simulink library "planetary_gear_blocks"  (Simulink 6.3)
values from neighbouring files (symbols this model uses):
  b_c = kb*J_c    (= 4.94590955184)    [architetture_epicicloidale.m]    (also in architetture_epicicloidale_cont.m; architetture_epicicloidale_HEV.m = 92.8974810391; architetture_epicicloidale_prova.m; architetture_HEV_controllo.m = 9.28974810391)
  b_p = kb*J_p    (= 8.12277148259)    [architetture_epicicloidale_HEV.m]    (also in architetture_HEV_controllo.m = 0.812277148259; architetture_HEV_startstop.m = 0.0731049433433; Confronto_CVT_EMR.m = 0; epicicloidale_confronto_statico_elastico.m)
  b_r = kb*J_r    (= 218.026030555)    [architetture_epicicloidale.m]    (also in architetture_epicicloidale_cont.m; architetture_epicicloidale_HEV.m; architetture_epicicloidale_prova.m; architetture_HEV_controllo.m = 21.8026030555)
  b_s = kb*J_s    (= 8.12277148259)    [architetture_epicicloidale.m]    (also in architetture_epicicloidale_cont.m; architetture_epicicloidale_HEV.m = 4.94590955184; architetture_epicicloidale_prova.m; architetture_HEV_controllo.m = 0.494590955184)
  d_cr = d0    (= 10)    [architetture_epicicloidale_HEV.m]    (also in architetture_HEV_controllo.m = 1000; architetture_HEV_startstop.m = 90; epicicloidale_confronto_statico_elastico.m; epicicloidale_statico.m)
  d_sc = d0    (= 10)    [architetture_epicicloidale_HEV.m]    (also in architetture_HEV_controllo.m = 1000; architetture_HEV_startstop.m = 90; epicicloidale_confronto_statico_elastico.m; epicicloidale_statico.m)
  J_c = 1.3*0.5*pi*rho_acc*hc*r_c^4    (= 0.0494590955184)    [architetture_epicicloidale.m]    (also in architetture_epicicloidale_cont.m; architetture_epicicloidale_HEV.m = 0.928974810391; architetture_epicicloidale_prova.m; architetture_HEV_controllo.m = 0.928974810391)
  J_p = Nr_sat*0.5*pi*rho_acc*(hs*r_p^4 + hc*r_p^4)    (= 0.0812277148259)    [architetture_epicicloidale_HEV.m]    (also in architetture_HEV_controllo.m; architetture_HEV_startstop.m; Confronto_CVT_EMR.m = 0; epicicloidale_confronto_statico_elastico.m)
  J_r = 0.5*pi*rho_acc*(hr*r_ri^4 + h_ring*(r_re^4-r_ri^4))    (= 2.18026030555)    [architetture_epicicloidale.m]    (also in architetture_epicicloidale_cont.m; architetture_epicicloidale_HEV.m; architetture_epicicloidale_prova.m; architetture_HEV_controllo.m)
  J_s = Nr_sat*0.5*pi*rho_acc*(hs*r_s^4 + hc*r_s^4)    (= 0.0812277148259)    [architetture_epicicloidale.m]    (also in architetture_epicicloidale_cont.m; architetture_epicicloidale_HEV.m = 0.0494590955184; architetture_epicicloidale_prova.m; architetture_HEV_controllo.m = 0.0494590955184)
  K_cr = K0    (= 10000)    [architetture_epicicloidale_HEV.m]    (also in architetture_HEV_controllo.m = 100000; architetture_HEV_startstop.m = 10000000; epicicloidale_confronto_statico_elastico.m; epicicloidale_statico.m)
  K_sc = K0    (= 10000)    [architetture_epicicloidale_HEV.m]    (also in architetture_HEV_controllo.m = 100000; architetture_HEV_startstop.m = 10000000; epicicloidale_confronto_statico_elastico.m; epicicloidale_statico.m)
  Nr_sat = 4    [architetture_epicicloidale.m]    (also in architetture_epicicloidale_cont.m; architetture_epicicloidale_HEV.m; architetture_epicicloidale_prova.m; architetture_HEV_controllo.m)
  r_p = xds*Np/(2*pi)    (= 0.0732112738223)    [architetture_epicicloidale_HEV.m]    (also in architetture_HEV_controllo.m; architetture_HEV_startstop.m; Confronto_CVT_EMR.m = 0.025; epicicloidale_confronto_statico_elastico.m)
  r_r = xds*Nr/(2*pi)    (= 0.248281711223)    [architetture_epicicloidale_HEV.m]    (also in architetture_HEV_controllo.m; architetture_HEV_startstop.m; Confronto_CVT_EMR.m = 0.1; epicicloidale_confronto_statico_elastico.m)
  r_s = xds*Ns/(2*pi)    (= 0.0732112738223)    [architetture_epicicloidale.m]    (also in architetture_epicicloidale_cont.m; architetture_epicicloidale_HEV.m = 0.101859163579; architetture_epicicloidale_prova.m; architetture_HEV_controllo.m = 0.101859163579)
  Tc = 0.05*ms    (= 5e-05)    [architetture_epicicloidale.m]    (also in architetture_epicicloidale_cont.m; architetture_epicicloidale_HEV.m; architetture_epicicloidale_prova.m; architetture_HEV_controllo.m)
  Tc_0 = 0*N*metri    (= 0)    [architetture_epicicloidale_HEV.m]    (also in architetture_HEV_controllo.m; architetture_HEV_startstop.m; epicicloidale_confronto_statico_elastico.m; epicicloidale_statico.m)
  Tr_0 = 0*N*metri    (= 0)    [architetture_epicicloidale_HEV.m]    (also in architetture_HEV_controllo.m; architetture_HEV_startstop.m; epicicloidale_confronto_statico_elastico.m; epicicloidale_statico.m)
  Ts_0 = 0*N*metri    (= 0)    [architetture_epicicloidale_HEV.m]    (also in architetture_HEV_controllo.m; architetture_HEV_startstop.m; epicicloidale_confronto_statico_elastico.m; epicicloidale_statico.m)
  Wc_0 = 0*0.1*rad/secondo    (= 0)    [architetture_epicicloidale.m]    (also in architetture_epicicloidale_cont.m; architetture_epicicloidale_HEV.m; architetture_epicicloidale_prova.m; Confronto_CVT_EMR.m)
  Wr_0 = Sys1.C(3,:)*[Wc_0; Wsc_0]    [architetture_epicicloidale.m]    (also in Confronto_CVT_EMR.m = 0; epicicloidale.m; epicicloidale_confronto_statico_elastico.m = [-r_s/r_r, 1+r_s/r_r]*[Ws_0; Wc_0]; epicicloidale_da_solo.m = [ -1/r_ri*r_c, (r_c+r_ri)/r_ri]*[Wc_0; Wsc_0])
  Ws_0 = 0.1*rad/secondo    (= 0.1)    [epicicloidale_confronto_statico_elastico.m]    (also in epicicloidale_statico.m; architetture_epicicloidale_statico.m = 0)
undefined symbols (not defined in the file or in its folder): Wr, Ws

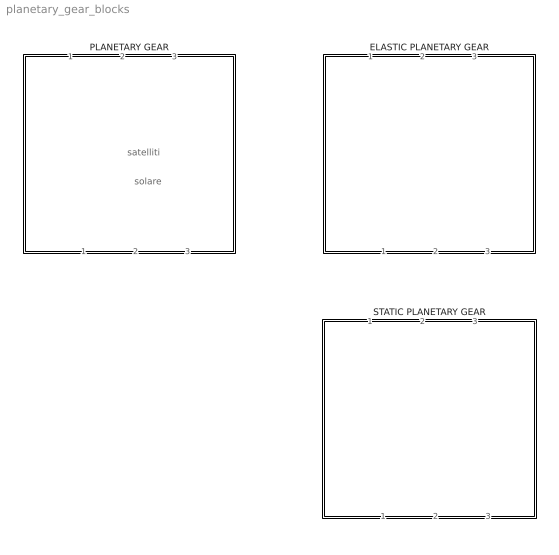
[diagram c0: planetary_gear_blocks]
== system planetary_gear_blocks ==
  note: solare
  note: satelliti
  ELASTIC PLANETARY GEAR : Subsystem  Orientation=down  mask(POG Gruppo epicicloidale){Par_solare=[J_s, b_s, r_s], Par_satelliti=[J_p, J_c, b_p, b_c, r_p, Nr_sat], Par_ring=[J_r, b_r, r_r], Solare_Satelliti=[K_sc, d_sc], Satelliti_Ring=[K_cr, d_cr], Cond_in=[Ts_0, Tc_0, Tr_0]}
      mask prompts: Par_solare "Parametri Solare: [J_s, b_s, r_s]-->[kg*m^2,N*m*s/rad,m]"; Par_satelliti "Parametri Satelliti: [J_p, J_c, b_p, b_c, r_p, Nr_sat]-->[kg*m^2,N*m*s/rad,m]"; Par_ring "Parametri Ring: [J_r, b_r, r_r]-->[kg*m^2,N*m*s/rad,m,m]"; Solare_Satelliti "Solare-Satelliti: [K_sc, d_sc]-->[N/m,N*m*s/rad]"; Satelliti_Ring "Satelliti-Ring: [K_cr, d_cr]-->[N/m,N*m*s/rad]"; Cond_in "Condizioni iniziali: [Ts_0, Tc_0, Tr_0]-->[N]"
      mask help: Gruppo epicicloidale: [J_s, J_p, J_c, J_r]= Inerzie di: solare, satelliti, porta-satelliti, ring; [b_s, b_p, b_c, b_r]= Attriti di: solare, satelliti, porta-satelliti, ring; [r_s, r_p, r_r]= Raggi di: solare, satelliti, ring; [Nr_sat]= Numero Satelliti; [K_sc, K_cr]= Elasticita' tra solare-satelliti e tra satelliti-ring; [d_sc, d_cr]= Elementi della matrice D; [Ws_0, Wc_0, Wr_0]=Velocita' iniziali di solare, porta-satelliti, ring;
      mask init:
      | J_s=double(Par_solare(1));          
      | b_s=double(Par_solare(2));            
      | r_s=double(Par_solare(3));           
      | %
      | J_p=double(Par_satelliti(1));            
      | J_c=double(Par_satelliti(2));            
      | b_p=double(Par_satelliti(3));            
      | b_c=double(Par_satelliti(4));            
      | r_p=double(Par_satelliti(5));            
      | Nr_sat=double(Par_satelliti(6));           
      | %
      | J_r=double(Par_ring(1));             
      | b_r=double(Par_ring(2));            
      | r_r=double(Par_ring(3));                  
      | %
      | %%%%%%%%%%%%%%%%%%%%%%%%%%%%%%%%%%%%%%%%%%%%%%%%%%%%%%%%%%%%%%%%%%%%%%%%%%%
      | %   Modello solo elastico
      | %%%%%%%%%%%%%%%%%%%%%%%%%%%%%%%%%%%%%%%%%%%%%%%%%%%%%%%%%%%%%%%%%%%%%%%%%%%
      |       
      |     %
      |     K_sc=double(Solare_Satelliti(1));
      |     d_sc=double(Solare_Satelliti(2));
      |     if(K_sc==0)
      |         K_sc=inf;
      |     end
      |     %
      |     K_cr=double(Satelliti_Ring(1));
      |     d_cr=double(Satelliti_Ring(2));
      |     if(K_cr==0)
      |         K_cr=inf;
      |     end
      |     
      |     %
      |     L=[1/K_sc,      0,      0;
      |             0,    J_p,      0;
      |             0,      0, 1/K_cr];
      |     %
      | 
      |     A=-[                          0,                        r_p,                          0;
      |                                -r_p, -d_sc*r_p^2-r_p^2*d_cr-b_p,                       -r_p;
      |                                   0,                        r_p,                          0];
      |        
      |     B=[                      r_s,                     -r_s,                        0;
      |                    -r_s*d_sc*r_p, -(d_cr*r_r-r_s*d_sc)*r_p,             r_p*d_cr*r_r;
      |                               0,                      r_r,                     -r_r];
      |     C=[                     r_s,            r_s*d_sc*r_p,                       0;
      |                            -r_s, (d_cr*r_r-r_s*d_sc)*r_p,                     r_r;
      |                               0,           -r_p*d_cr*r_r,                    -r_r];
      |     
      |     D= [    b_s+r_s^2*d_sc,               -r_s^2*d_sc,                         0;
      |                -r_s^2*d_sc, b_c+r_s^2*d_sc+r_r^2*d_cr,               -r_r^2*d_cr;
      |                          0,               -r_r^2*d_cr,            b_r+r_r^2*d_cr];
      |        
      |      %
      |     Ts_0=double(Cond_in(1));
      |     Tc_0=double(Cond_in(2));
      |     Tr_0=double(Cond_in(3));
      |     
      |     %
      |     We_0=[Ts_0 Tc_0 Tr_0];
  PLANETARY GEAR : Subsystem  Orientation=down  mask(POG Gruppo epicicloidale){Par_solare=[J_s, b_s, r_s], Par_satelliti=[J_p, J_c, b_p, b_c, r_p, Nr_sat], Par_ring=[J_r, b_r, r_r], Tipo_di_Modello=Modello esteso, Cond_in_Ws_Wc=[Ws_0,  Wc_0], Cond_in_Wc_Wr=[Wc_0,  Wr_0], Cond_in_Ws_Wr=[Ws_0,  Wr_0], Solare_Satelliti=[K_sc, d_sc], Satelliti_Ring=[K_cr, d_cr], Cond_in=[Ws_0, Wc_0, Wr_0]}
      mask prompts: Par_solare "Parametri Solare: [J_s, b_s, r_s]-->[kg*m^2,N*m*s/rad,m]"; Par_satelliti "Parametri Satelliti: [J_p, J_c, b_p, b_c, r_p, Nr_sat]-->[kg*m^2,N*m*s/rad,m]"; Par_ring "Parametri Ring: [J_r, b_r, r_r]-->[kg*m^2,N*m*s/rad,m,m]"; Tipo_di_Modello "Tipo di modello"; Cond_in_Ws_Wc "Condizioni iniziali: [Ws_0,  Wc_0]-->[rad/s]"; Cond_in_Wc_Wr "Condizioni iniziali: [Wc_0,  Wr_0]-->[rad/s]"; Cond_in_Ws_Wr "Condizioni iniziali: [Ws_0,  Wr_0]-->[rad/s]"; Solare_Satelliti "Solare-Satelliti: [K_sc, d_sc]-->[N/m,N*m*s/rad]"; Satelliti_Ring "Satelliti-Ring: [K_cr, d_cr]-->[N/m,N*m*s/rad]"; Cond_in "Condizioni iniziali: [Ws_0,  Wc_0, Wr_0]-->[rad/s]"
      mask help: Gruppo epicicloidale: [J_s, J_p, J_c, J_r]= Inerzie di: solare, satelliti, porta-satelliti, ring; [b_s, b_p, b_c, b_r]= Attriti di: solare, satelliti, porta-satelliti, ring; [r_s, r_p, r_r]= Raggi di: solare, satelliti, ring; [Nr_sat]= Numero Satelliti; [K_sc, K_cr]= Elasticita' tra solare-satelliti e tra satelliti-ring; [d_sc, d_cr]= Elementi della matrice D; [Ws_0, Wc_0, Wr_0]=Velocita' iniziali di solare, porta-satelliti, ring;
      mask init:
      | J_s=double(Par_solare(1));          
      | b_s=double(Par_solare(2));            
      | r_s=double(Par_solare(3));           
      | %
      | J_p=double(Par_satelliti(1));            
      | J_c=double(Par_satelliti(2));            
      | b_p=double(Par_satelliti(3));            
      | b_c=double(Par_satelliti(4));            
      | r_p=double(Par_satelliti(5));            
      | Nr_sat=double(Par_satelliti(6));           
      | %
      | J_r=double(Par_ring(1));             
      | b_r=double(Par_ring(2));            
      | r_r=double(Par_ring(3));                  
      | %
      | %%%%%%%%%%%%%%%%%%%%%%%%%%%%%%%%%%%%%%%%%%%%%%%%%%%%%%%%%%%%%%%%%%%%%%%%%%%
      | %   Modello esteso e modelli ridotti
      | %%%%%%%%%%%%%%%%%%%%%%%%%%%%%%%%%%%%%%%%%%%%%%%%%%%%%%%%%%%%%%%%%%%%%%%%%%%
      | if Tipo_di_Modello=='Modello esteso       '
      |     %
      |     K_sc=double(Solare_Satelliti(1));
      |     d_sc=double(Solare_Satelliti(2));
      |     if(K_sc==0)
      |         K_sc=inf;
      |     end
      |     %
      |     K_cr=double(Satelliti_Ring(1));
      |     d_cr=double(Satelliti_Ring(2));
      |     if(K_cr==0)
      |         K_cr=inf;
      |     end
      |     %
      |     %
      |     L=[ J_s,    0,      0,      0,      0,      0;
      |         0, 1/K_sc,      0,      0,      0,      0;
      |         0,      0,    J_p,      0,      0,      0;
      |         0,      0,      0,    J_c,      0,      0;
      |         0,      0,      0,      0, 1/K_cr,      0;
      |         0,      0,      0,      0,      0,    J_r];
      |     %
      |     A=- [-b_s-r_s^2*d_sc,                       -r_s,              -r_s*d_sc*r_p,                 r_s^2*d_sc,                          0,                          0;
      |                         r_s,                          0,                        r_p,                       -r_s,                          0,                          0;
      |               -r_s*d_sc*r_p,                       -r_p, -b_p-d_sc*r_p^2-d_cr*r_p^2,  r_s*d_sc*r_p-d_cr*r_p*r_r,                       -r_p,               d_cr*r_p*r_r;
      |                  r_s^2*d_sc,                        r_s,  r_s*d_sc*r_p-d_cr*r_p*r_r, -b_c-r_s^2*d_sc-d_cr*r_r^2,                       -r_r,                 d_cr*r_r^2;
      |                           0,                          0,                        r_p,                        r_r,                          0,                       -r_r;
      |                           0,                          0,               d_cr*r_p*r_r,                 d_cr*r_r^2,                        r_r,            -b_r-d_cr*r_r^2];
      | %                         
      |     B=[ 1, 0, 0;
      |         0, 0, 0;
      |         0, 0, 0;
      |         0, 1, 0;
      |         0, 0, 0;
      |         0, 0, 1];
      |     %
      |     C=[ 1, 0, 0, 0, 0, 0;
      |         0, 0, 0, 1, 0, 0;
      |         0, 0, 0, 0, 0, 1];
      |     %
      |     Ws_0=double(Cond_in(1));
      |     Wc_0=double(Cond_in(2));
      |     Wr_0=double(Cond_in(3));
      |     Wp_0=r_s*(Wc_0-Ws_0)/r_p;
      |     Wpc_0=[Wp_0 Wc_0];
      |     %
      |     We_0=[Ws_0 0 Wpc_0 0 Wr_0 ];
      |     %
      | elseif Tipo_di_Modello=='Modello ridotto Ws-Wc'
      |     L = [(J_s*r_p^2*r_r^2+r_s^2*J_p*r_r^2+r_s^2*J_r*r_p^2)/r_p^2/r_r^2,                                      -r_s*(r_s*J_p*r_r^2+J_r*r_p^2*r_s+J_r*r_p^2*r_r)/r_p^2/r_r^2;
      |            -r_s*(r_s*J_p*r_r^2+J_r*r_p^2*r_s+J_r*r_p^2*r_r)/r_p^2/r_r^2, (J_c*r_p^2*r_r^2+r_s^2*J_p*r_r^2+r_s^2*J_r*r_p^2+2*J_r*r_p^2*r_s*r_r+J_r*r_p^2*r_r^2)/r_p^2/r_r^2];
      |     %
      |     A=-[ -(b_s*r_p^2*r_r^2+r_s^2*b_p*r_r^2+r_s^2*b_r*r_p^2)/r_p^2/r_r^2,                                        r_s*(r_s*b_p*r_r^2+b_r*r_p^2*r_s+b_r*r_p^2*r_r)/r_p^2/r_r^2;
      |         r_s*(r_s*b_p*r_r^2+b_r*r_p^2*r_s+b_r*r_p^2*r_r)/r_p^2/r_r^2, -(b_c*r_p^2*r_r^2+r_s^2*b_p*r_r^2+r_s^2*b_r*r_p^2+2*b_r*r_p^2*r_s*r_r+b_r*r_p^2*r_r^2)/r_p^2/r_r^2];
      |     %
      |     B= [  1,             0,    -1/r_r*r_s;
      |            0,             1, (r_s+r_r)/r_r];
      |     %
      |     C= [            1,               0;
      |                     0,               1;
      |            -1/r_r*r_s, (r_s+r_r)/r_r];
      |     %
      |     Ws_0=double(Cond_in_Ws_Wc(1));
      |     Wc_0=double(Cond_in_Ws_Wc(2));
      |     We_0=[Ws_0 Wc_0];
      |     %
      | elseif Tipo_di_Modello=='Modello ridotto Wc-Wr'
      |     L= [ (J_c*r_s^2*r_p^2+J_s*r_p^2*r_s^2+2*J_s*r_p^2*r_s*r_r+J_s*r_p^2*r_r^2+r_r^2*J_p*r_s^2)/r_s^2/r_p^2,                                      -r_r*(J_s*r_p^2*r_s+J_s*r_p^2*r_r+r_r*J_p*r_s^2)/r_s^2/r_p^2;
      |           -r_r*(J_s*r_p^2*r_s+J_s*r_p^2*r_r+r_r*J_p*r_s^2)/r_s^2/r_p^2,                                     (J_r*r_s^2*r_p^2+J_s*r_p^2*r_r^2+r_r^2*J_p*r_s^2)/r_s^2/r_p^2];
      | 
      |     A=-[  -(b_c*r_s^2*r_p^2+b_s*r_p^2*r_s^2+2*b_s*r_p^2*r_s*r_r+b_s*r_p^2*r_r^2+r_r^2*b_p*r_s^2)/r_s^2/r_p^2,                                        r_r*(b_s*r_p^2*r_s+b_s*r_p^2*r_r+r_r*b_p*r_s^2)/r_s^2/r_p^2;
      |          r_r*(b_s*r_p^2*r_s+b_s*r_p^2*r_r+r_r*b_p*r_s^2)/r_s^2/r_p^2,                                     -(b_r*r_s^2*r_p^2+b_s*r_p^2*r_r^2+r_r^2*b_p*r_s^2)/r_s^2/r_p^2];
      | 
      |     B= [ (r_s+r_r)/r_s,    1,   0;
      |             -1/r_s*r_r,    0,   1];
      | 
      |     C= [ (r_s+r_r)/r_s,    -1/r_s*r_r;
      |                       1,            0;
      |                       0,            1];
      |     %
      |     Wc_0=double(Cond_in_Wc_Wr(1));
      |     Wr_0=double(Cond_in_Wc_Wr(2));
      |     We_0=[Wc_0 Wr_0];
      |     %
      | elseif Tipo_di_Modello=='Modello ridotto Ws-Wr'
      |     L= [ (J_c*r_s^2*r_p^2+J_s*r_p^2*r_s^2+2*J_s*r_p^2*r_s*r_r+J_s*r_p^2*r_r^2+r_r^2*J_p*r_s^2)/r_p^2/(r_s+r_r)^2,                                                      -r_s*r_r*(r_r*J_p*r_s-J_c*r_p^2)/r_p^2/(r_s+r_r)^2;
      |           -r_s*r_r*(r_r*J_p*r_s-J_c*r_p^2)/r_p^2/(r_s+r_r)^2, (J_r*r_s^2*r_p^2+2*J_r*r_p^2*r_s*r_r+J_r*r_p^2*r_r^2+r_r^2*J_p*r_s^2+r_r^2*J_c*r_p^2)/r_p^2/(r_s+r_r)^2];
      | 
      |     A=-[-(b_c*r_s^2*r_p^2+b_s*r_p^2*r_s^2+2*b_s*r_p^2*r_s*r_r+b_s*r_p^2*r_r^2+r_r^2*b_p*r_s^2)/r_p^2/(r_s+r_r)^2,                                                      -r_s*r_r*(-r_s*r_r*b_p+r_p^2*b_c)/r_p^2/(r_s+r_r)^2;
      |                                                               -r_s*r_r*(-r_s*r_r*b_p+r_p^2*b_c)/r_p^2/(r_s+r_r)^2, -(b_r*r_p^2*r_s^2+2*b_r*r_p^2*r_s*r_r+b_r*r_p^2*r_r^2+r_r^2*b_p*r_s^2+r_r^2*r_p^2*b_c)/r_p^2/(r_s+r_r)^2];
      | 
      |     B=[   1,  1/(r_s+r_r)*r_s, 0;
      |           0, 1/(r_s+r_r)*r_r, 1];
      | 
      |     C=[                 1,                  0;
      |          1/(r_s+r_r)*r_s, 1/(r_s+r_r)*r_r;
      |                         0,                  1];
      |     Ws_0=double(Cond_in_Ws_Wr(1));
      |     Wr_0=double(Cond_in_Ws_Wr(2));
      |     We_0=[Ws_0 Wr_0];
      | end
  STATIC PLANETARY GEAR : Subsystem  Orientation=down  AncestorBlock=|  mask(POG Gruppo epicicloidale){Raggi_sun_ring=[r_s, r_r], Tipo_di_Modello=Ws-Tc-Wr, Cond_in_Ws_Wc=[Ws_0,  Wc_0], Cond_in_Wc_Wr=[Wc_0,  Wr_0], Cond_in_Ws_Wr=[Ws_0,  Wr_0], Cond_in=[Ws_0, Wc_0, Wr_0]}
      | planetary_gear_blocks/STATIC
      | PLANETARY
      | GEAR
      mask prompts: Raggi_sun_ring "Raggi Sun, Ring: [r_s, r_r]-->[m,m]"; Tipo_di_Modello "Ingressi:"; Cond_in_Ws_Wc "Condizioni iniziali: [Ws_0,  Wc_0]-->[rad/s]"; Cond_in_Wc_Wr "Condizioni iniziali: [Wc_0,  Wr_0]-->[rad/s]"; Cond_in_Ws_Wr "Condizioni iniziali: [Ws_0,  Wr_0]-->[rad/s]"; Cond_in "Condizioni iniziali: [Ws_0,  Wc_0, Wr_0]-->[rad/s]"
      mask help: Gruppo epicicloidale: [r_s, r_r]= Raggi di: sun e ring; [Ws_0, Wc_0, Wr_0]=Velocita' iniziali di sun, carrier, ring;
      mask init:
      | r_s=Raggi_sun_ring(1);
      | r_r=Raggi_sun_ring(2);
      | 
      | %
      | %%%%%%%%%%%%%%%%%%%%%%%%%%%%%%%%%%%%%%%%%%%%%%%%%%%%%%%%%%%%%%%%%%%%%%%%%%%
      | %   Modello statico tutti i casi
      | %%%%%%%%%%%%%%%%%%%%%%%%%%%%%%%%%%%%%%%%%%%%%%%%%%%%%%%%%%%%%%%%%%%%%%%%%%%
      | if Tipo_di_Modello=='Ws-Wc-Tr'
      |       %
      |     B= [         0,             0,   -1/r_r*r_s;
      |                  0,             0,   (r_s+r_r)/r_r;
      |         -1/r_r*r_s, (r_s+r_r)/r_r,              0];
      |     %
      |     Ws_0=double(Cond_in_Ws_Wc(1));
      |     Wc_0=double(Cond_in_Ws_Wc(2));
      |     We_0=[Ws_0 Wc_0];
      |     %
      | elseif Tipo_di_Modello=='Ts-Wc-Wr'
      |     B= [            0,  (r_s+r_r)/r_s,  -1/r_s*r_r;
      |         (r_s+r_r)/r_s,              0,           0;
      |            -1/r_s*r_r,              0,           0];
      |    %
      |     Wc_0=double(Cond_in_Wc_Wr(1));
      |     Wr_0=double(Cond_in_Wc_Wr(2));
      |     We_0=[Wc_0 Wr_0];
      |     %
      | elseif Tipo_di_Modello=='Ws-Tc-Wr'
      |  
      |     B=[              0,  1/(r_s+r_r)*r_s,               0;
      |        1/(r_s+r_r)*r_s,                0, 1/(r_s+r_r)*r_r;
      |                      0,  1/(r_s+r_r)*r_r,               0];
      |    %
      |     Ws_0=double(Cond_in_Ws_Wr(1));
      |     Wr_0=double(Cond_in_Ws_Wr(2));
      |     We_0=[Ws_0 Wr_0];
      | end

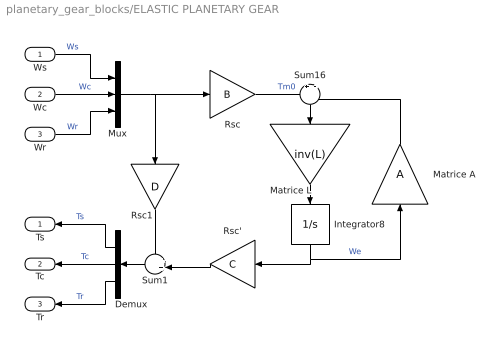
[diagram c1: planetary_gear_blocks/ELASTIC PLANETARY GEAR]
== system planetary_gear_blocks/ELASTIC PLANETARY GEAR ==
  Ws : Inport
  Wc : Inport  Port=2
  Wr : Inport  Port=3
  Demux : Demux  Orientation=left  Outputs=3
  Integrator8 : Integrator  Orientation=down  InitialCondition=We_0  LowerSaturationLimit=0
  Matrice A : Gain  Orientation=up  Gain=A  Multiplication=Matrix(K*u)
  Matrice L : Gain  Orientation=down  Gain=inv(L)  Multiplication=Matrix(K*u)
  Mux : Mux  Inputs=3
  Rsc : Gain  Gain=B  Multiplication=Matrix(K*u)
  Rsc' : Gain  Orientation=left  Gain=C  Multiplication=Matrix(K*u)
  Rsc1 : Gain  Orientation=down  Gain=D  Multiplication=Matrix(K*u)
  Sum1 : Sum  Orientation=left  Inputs=++|
  Sum16 : Sum  Orientation=down  Inputs=+|-
  Ts : Outport  Orientation=left
  Tc : Outport  Orientation=left  Port=2
  Tr : Outport  Orientation=left  Port=3
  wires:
  Demux/3 -> Tr/1  "Tr"
  Demux/2 -> Tc/1  "Tc"
  Demux/1 -> Ts/1  "Ts"
  Mux/1 -> Rsc/1, Rsc1/1
  Wr/1 -> Mux/3  "Wr"
  Wc/1 -> Mux/2  "Wc"
  Ws/1 -> Mux/1  "Ws"
  Matrice A/1 -> Sum16/2
  Integrator8/1 -> Rsc'/1, Matrice A/1  "We"
  Matrice L/1 -> Integrator8/1
  Sum16/1 -> Matrice L/1
  Rsc/1 -> Sum16/1  "Tm0"
  Rsc'/1 -> Sum1/2
  Sum1/1 -> Demux/1
  Rsc1/1 -> Sum1/1

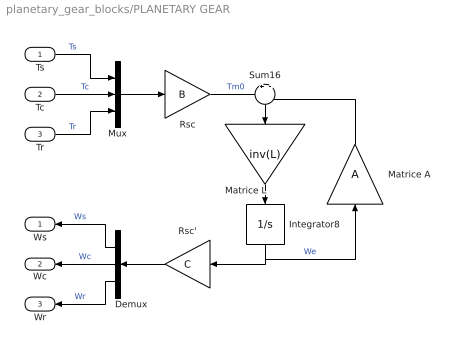
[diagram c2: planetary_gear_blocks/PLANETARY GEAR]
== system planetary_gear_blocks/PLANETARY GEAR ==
  Ts : Inport
  Tc : Inport  Port=2
  Tr : Inport  Port=3
  Demux : Demux  Orientation=left  Outputs=3
  Integrator8 : Integrator  Orientation=down  InitialCondition=We_0  LowerSaturationLimit=0
  Matrice A : Gain  Orientation=up  Gain=A  Multiplication=Matrix(K*u)
  Matrice L : Gain  Orientation=down  Gain=inv(L)  Multiplication=Matrix(K*u)
  Mux : Mux  Inputs=3
  Rsc : Gain  Gain=B  Multiplication=Matrix(K*u)
  Rsc' : Gain  Orientation=left  Gain=C  Multiplication=Matrix(K*u)
  Sum16 : Sum  Orientation=down  Inputs=+|-
  Ws : Outport  Orientation=left
  Wc : Outport  Orientation=left  Port=2
  Wr : Outport  Orientation=left  Port=3
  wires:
  Rsc/1 -> Sum16/1  "Tm0"
  Sum16/1 -> Matrice L/1
  Matrice L/1 -> Integrator8/1
  Integrator8/1 -> Matrice A/1, Rsc'/1  "We"
  Matrice A/1 -> Sum16/2
  Ts/1 -> Mux/1  "Ts"
  Tc/1 -> Mux/2  "Tc"
  Tr/1 -> Mux/3  "Tr"
  Mux/1 -> Rsc/1
  Rsc'/1 -> Demux/1
  Demux/1 -> Ws/1  "Ws"
  Demux/2 -> Wc/1  "Wc"
  Demux/3 -> Wr/1  "Wr"

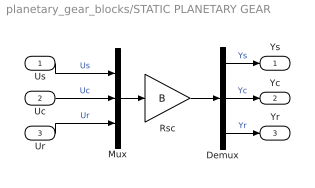
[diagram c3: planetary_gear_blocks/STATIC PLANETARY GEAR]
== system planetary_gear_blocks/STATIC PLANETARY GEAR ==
  Us : Inport
  Uc : Inport  Port=2
  Ur : Inport  Port=3
  Demux : Demux  Outputs=3
  Mux : Mux  Inputs=3
  Rsc : Gain  Gain=B  Multiplication=Matrix(K*u)
  Ys : Outport
  Yc : Outport  Port=2
  Yr : Outport  Port=3
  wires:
  Us/1 -> Mux/1  "Us"
  Uc/1 -> Mux/2  "Uc"
  Mux/1 -> Rsc/1
  Demux/1 -> Ys/1  "Ys"
  Demux/2 -> Yc/1  "Yc"
  Ur/1 -> Mux/3  "Ur"
  Demux/3 -> Yr/1  "Yr"
  Rsc/1 -> Demux/1
